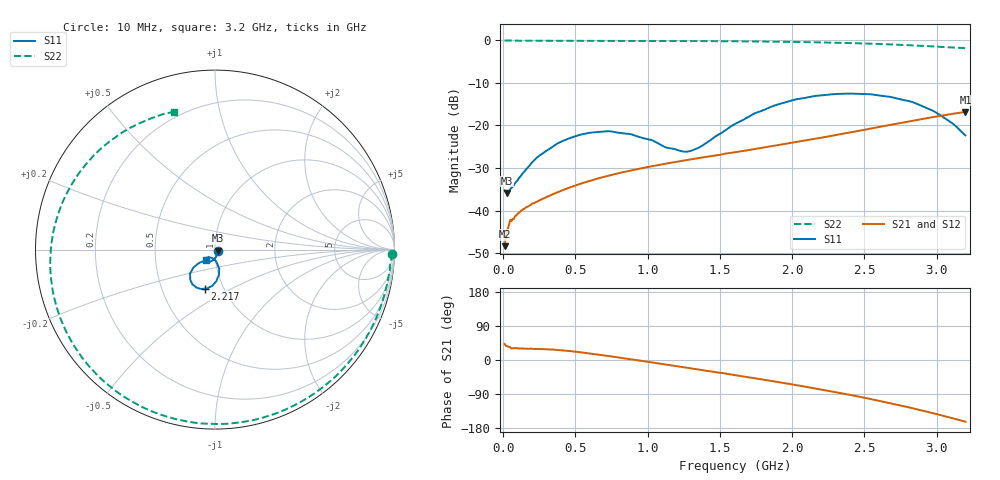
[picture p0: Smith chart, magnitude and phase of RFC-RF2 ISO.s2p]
!Agilent Technologies,N5230A,MY45001650,A.07.50.48
!Agilent N5230A: A.07.50.48
!Date: Monday, December 05, 2022 16:06:33
!Correction: S11(Full 2 Port(1,2))
!S21(Full 2 Port(1,2))
!S12(Full 2 Port(1,2))
!S22(Full 2 Port(1,2))
!S2P File: Measurements: S11, S21, S12, S22:
# Hz S  dB  R 50
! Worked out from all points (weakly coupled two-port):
!   400 points, 10 MHz to 3.2 GHz, reference 50 ohm
!   highest |S21| = -16.86 dB at 3.2 GHz (marker M1); lowest = -48.3 dB at 10 MHz (marker M2)
!   lowest |S11| = -35.9 dB at 25.99 MHz (marker M3), VSWR 1.03, Z = 51.5 - j0.604 ohm
!   |S11| at or under -10 dB: start of sweep to end of sweep
!   |S22| runs from -1.9 to -0.1 dB; largest |S21 - S12| = 0.00028
!   S11 on the Smith chart (normalised r, x): 10 MHz: 1.03, -0.01; 2.217 GHz: 0.82, -0.37; 3.2 GHz: 0.90, -0.11
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1e7  -35.24 -19.6  -48.31 42.5  -47.90 44.7  -0.13 -1.3
1.799499e7  -35.60 -19.6  -45.97 37.7  -46.23 38.8  -0.14 -1.8
2.598997e7  -35.87 -21.3  -44.93 36.5  -45.07 36.8  -0.13 -2.5
4.997494e7  -34.95 -27.1  -42.10 33.3  -42.08 32.9  -0.18 -4.8
5.796992e7  -34.61 -35.9  -42.42 30.1  -42.15 29.1  -0.18 -5.4
1.219298e8  -31.89 -60.8  -40.05 30.1  -40.00 29.9  -0.19 -11.0
2.258647e8  -27.81 -82.3  -37.98 29.1  -38.01 29.3  -0.21 -20.4
2.978195e8  -26.01 -92.5  -36.85 28.3  -36.84 28.5  -0.22 -26.6
5.456642e8  -22.12 -117.3  -33.57 19.9  -33.57 19.8  -0.22 -47.8
7.455388e8  -21.43 -129.7  -31.66 9.6  -31.67 9.6  -0.23 -64.0
8.894486e8  -22.13 -135.7  -30.54 1.6  -30.54 1.6  -0.24 -75.1
1.081328e9  -24.41 -133.3  -29.25 -9.4  -29.26 -9.4  -0.25 -89.3
1.297193e9  -26.02 -104.4  -27.99 -21.9  -27.99 -22.0  -0.27 -104.4
1.608997e9  -19.61 -77.6  -26.28 -40.3  -26.28 -40.3  -0.33 -124.9
1.872832e9  -15.43 -86.4  -24.83 -56.3  -24.83 -56.2  -0.42 -141.8
2.136667e9  -13.25 -100.2  -23.30 -73.4  -23.30 -73.4  -0.54 -159.0
2.216617e9  -12.96 -104.6  -22.81 -78.9  -22.82 -78.8  -0.59 -164.4
2.456466e9  -12.64 -118.4  -21.33 -96.2  -21.33 -96.2  -0.79 178.3
2.672331e9  -13.31 -129.8  -19.96 -113.3  -19.96 -113.3  -1.04 161.0
2.824236e9  -14.47 -136.6  -19.00 -126.4  -19.00 -126.4  -1.28 147.3
2.97614e9  -16.61 -140.3  -18.08 -140.5  -18.08 -140.5  -1.54 132.0
3.2e9  -22.36 -128.5  -16.86 -162.8  -16.86 -162.8  -1.93 106.5
